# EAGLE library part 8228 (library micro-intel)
MICROCOMPUTER/PERIPHERAL DEVICE
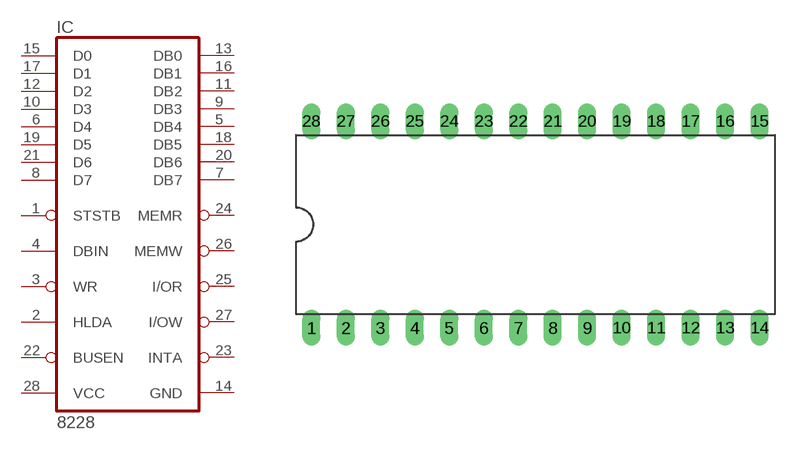
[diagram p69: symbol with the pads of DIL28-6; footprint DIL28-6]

Designator prefix IC

## 8228 (OC_FARNELL: unknown; OC_NEWARK: unknown)  [DIL28-6]
1  STSTB  in
2  HLDA  in
3  WR  in
4  DBIN  in
5  DB4
6  D4
7  DB7
8  D7
9  DB3
10  D3
11  DB2
12  D2
13  DB0
14  GND  pwr
15  D0
16  DB1
17  D1
18  DB5
19  D5
20  DB6
21  D6
22  BUSEN  in
23  INTA  out
24  MEMR  out
25  I/OR  out
26  MEMW  out
27  I/OW  out
28  VCC  pwr

## Footprint DIL28-6 (pad centres in mm)
Dual In Line Package 0.6 inch
drill 0.813 long: 1 -16.51,-7.62; 2 -13.97,-7.62; 3 -11.43,-7.62; 4 -8.89,-7.62; 5 -6.35,-7.62; 6 -3.81,-7.62; 7 -1.27,-7.62; 8 1.27,-7.62; 9 3.81,-7.62; 10 6.35,-7.62; 11 8.89,-7.62; 12 11.43,-7.62; 13 13.97,-7.62; 14 16.51,-7.62; 15 16.51,7.62; 16 13.97,7.62; 17 11.43,7.62; 18 8.89,7.62; 19 6.35,7.62; 20 3.81,7.62; 21 1.27,7.62; 22 -1.27,7.62; 23 -3.81,7.62; 24 -6.35,7.62; 25 -8.89,7.62; 26 -11.43,7.62; 27 -13.97,7.62; 28 -16.51,7.62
